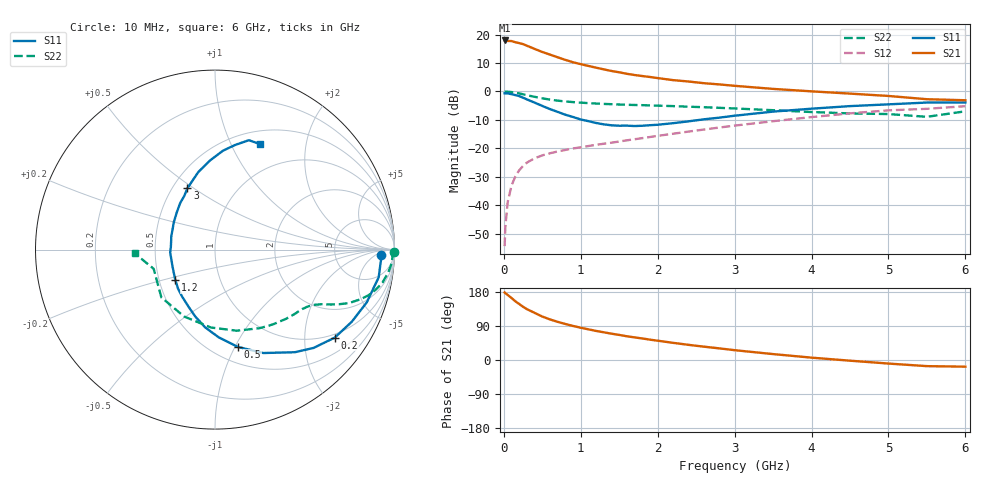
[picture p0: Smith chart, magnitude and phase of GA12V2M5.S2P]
! Infineon Technologies  Discrete & RF Semiconductors
! BF775
! Si NPN RF Bipolar Junction Transistor in SOT23
! VCE = 12 V  IC = 2.5 mA
! Common Emitter S-Parameters:  May  1996
# GHz  S  MA  R  50
!  f  S11  S21  S12  S22
! GHz  MAG  ANG  MAG  ANG  MAG  ANG  MAG  ANG
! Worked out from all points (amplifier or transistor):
!   36 points, 10 MHz to 6 GHz, reference 50 ohm
!   highest |S21| = 17.9 dB at 10 MHz (marker M1)
!   |S21| within 3 dB of that: start of sweep to 402.7 MHz
!   unconditionally stable (mu >= 1): 1.157 GHz to 3.056 GHz
!   at 250 MHz: K = 0.32, MSG = 21.4 dB, |S12| = -26.2 dB
!   at 1.4 GHz: K = 1.08, MAG = 10.8 dB, |S12| = -18.0 dB
!   at 6 GHz: K = 0.90, MSG = 1.0 dB, |S12| = -5.2 dB
!   S11 on the Smith chart (normalised r, x): 10 MHz: 22, -10; 200 MHz: 0.90, -2.79; 500 MHz: 0.65, -1.03; 1.2 GHz: 0.61, -0.22; 3 GHz: 0.59, +0.47; 6 GHz: 0.65, +1.29
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0.01  0.9274 -1.9  7.885 178.2  0.0019 82.4  0.9973 -0.7
0.02  0.9263 -3.7  7.814 176.3  0.0042 85.6  0.9889 -1.5
0.05  0.925 -9.6  7.735 171.6  0.0113 83.7  0.9896 -3.9
0.1  0.8951 -19.2  7.69 163.5  0.0222 78.8  0.9739 -7.5
0.15  0.8616 -27.8  7.336 154.9  0.0321 74.0  0.9507 -11.2
0.2  0.8281 -36.3  7.08 147.7  0.0411 69.8  0.9243 -13.9
0.25  0.7759 -44.9  6.792 140.4  0.049 65.6  0.8915 -16.6
0.3  0.7246 -52.1  6.372 134.2  0.0561 62.7  0.8594 -18.7
0.4  0.6358 -65.0  5.601 124.4  0.0668 58.0  0.8049 -21.7
0.5  0.5568 -76.8  4.942 114.6  0.0751 55.2  0.7569 -23.7
0.6  0.4892 -87.6  4.444 107.1  0.0817 52.8  0.7183 -25.2
0.7  0.4368 -97.2  3.989 100.6  0.0881 51.8  0.6889 -26.3
0.8  0.3893 -106.3  3.588 95.0  0.0936 51.0  0.6659 -27.2
1.1  0.3003 -133.2  2.809 80.9  0.1096 51.5  0.623 -30.0
1.2  0.2785 -142.6  2.617 76.7  0.1151 51.8  0.6124 -30.9
1.6  0.2504 -176.2  2.043 62.6  0.1382 53.4  0.5826 -35.3
2.2  0.2765 145.9  1.581 45.3  0.1805 54.4  0.5524 -44.3
3  0.3743 114.3  1.256 25.9  0.2506 52.0  0.5022 -60.8
3.5  0.4418 102.2  1.109 15.6  0.2996 48.1  0.4679 -75.0
4.5  0.5522 85.5  0.916 -1.8  0.4117 37.2  0.4106 -114.7
5.5  0.6381 72.8  0.73 -16.2  0.4947 20.8  0.358 -162.6
6  0.6391 67.0  0.7 -17.6  0.5506 16.2  0.4475 -177.3
